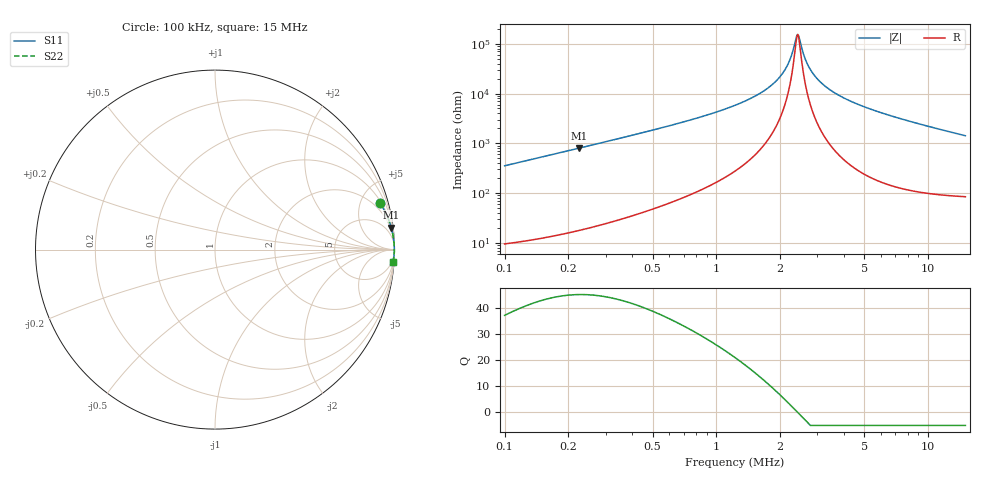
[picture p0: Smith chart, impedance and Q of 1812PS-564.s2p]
# MHz S MA R 50
!Freq  MagS11  AngS11  MagS21  AngS21  MagS12  AngS12  MagS22  AngS22
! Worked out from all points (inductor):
!   801 points, 100 kHz to 15 MHz, reference 50 ohm
!   read as one part in series: L = 560 uH near 102.5 kHz
!   highest Q = 45.1 at 224.3 kHz (marker M1), where L = 565 uH
!   self-resonance near 2.409 MHz
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0.1  0.9553 15.7  0.271 -72.7  0.271 -72.7  0.9553 15.7
0.1560013  0.98 10.2  0.1778 -78.4  0.1778 -78.4  0.98 10.2
0.2243338  0.9895 7.1  0.1243 -81.6  0.1243 -81.6  0.9895 7.1
0.3868518  0.9958 4.1  0.0713 -84.5  0.0713 -84.5  0.9958 4.1
0.6149405  0.9979 2.5  0.04316 -85.9  0.04316 -85.9  0.9979 2.5
1.603284  0.9992 0.6  0.009978 -85.2  0.009978 -85.2  0.9992 0.6
1.946857  0.9993 0.3  0.005208 -82.2  0.005208 -82.2  0.9993 0.3
2.179195  0.9993 0.1  0.002571 -74.9  0.002571 -74.9  0.9993 0.1
2.262647  0.9993 0.1  0.001729 -67.5  0.001729 -67.5  0.9993 0.1
2.364055  0.9993 0.0  0.0008668 -41.1  0.0008668 -41.1  0.9993 0.0
2.408895  0.9993 0.0  0.000664 -11.2  0.000664 -11.2  0.9993 0.0
2.470008  0.9994 -0.0  0.0007946 35.2  0.0007946 35.2  0.9994 -0.0
2.596924  0.9994 -0.1  0.001757 68.3  0.001757 68.3  0.9994 -0.1
2.713314  0.9994 -0.2  0.002744 76.2  0.002744 76.2  0.9994 -0.2
2.870656  0.9993 -0.2  0.004054 80.6  0.004054 80.6  0.9993 -0.2
3.336291  0.9993 -0.4  0.007664 84.6  0.007664 84.6  0.9993 -0.4
4.051235  0.9992 -0.7  0.01262 86.1  0.01262 86.1  0.9992 -0.7
5.075882  0.999 -1.1  0.01898 86.4  0.01898 86.4  0.999 -1.1
7.578772  0.9981 -1.9  0.0329 85.8  0.0329 85.8  0.9981 -1.9
10.04625  0.9969 -2.6  0.04568 84.8  0.04568 84.8  0.9969 -2.6
12.58717  0.9953 -3.3  0.05839 83.7  0.05839 83.7  0.9953 -3.3
15  0.9934 -4.0  0.0702 82.6  0.0702 82.6  0.9934 -4.0
